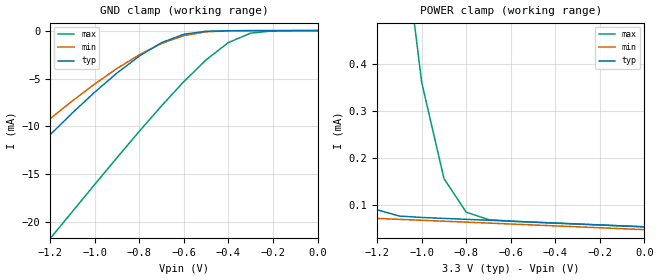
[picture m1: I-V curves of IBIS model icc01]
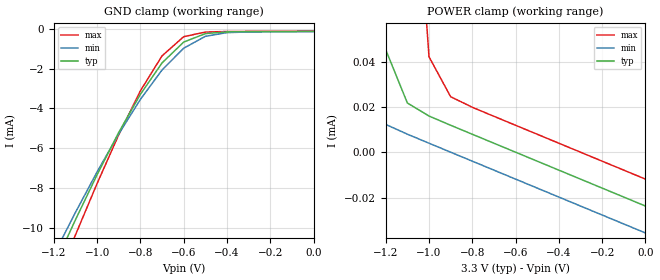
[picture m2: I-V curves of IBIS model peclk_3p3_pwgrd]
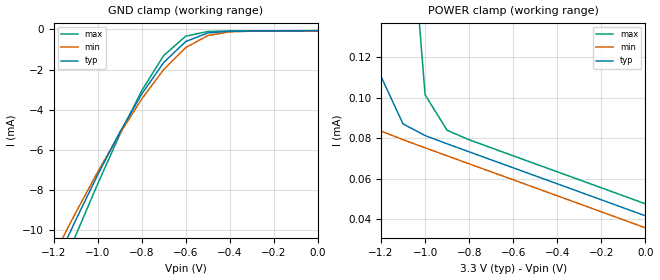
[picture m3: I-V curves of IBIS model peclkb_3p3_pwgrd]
[IBIS ver]   2.1
[File name]   mpc941v2.ibs
[File Rev]   2.2 {April 29, 2002}
[Date]   February 5th, 2002
[Disclaimer]   This information is for modeling purposes only
|   and is not guaranteed.
[Source]   Timing Solutions Operations
[Copyright]   Copyright 2001, Motorola Incorporated,
|   all rights reserved.
[Component]   MPC9413p3
[Manufacturer]   Motorola
[Package]
|   typ   min   max
R_pkg   0.048   .038   0.053
L_pkg   6.045nH   5.084nH   7.950nH
C_pkg   0.813pF   0.560pF   1.157pF
[Pin]   signal_name model_name R_pin L_pin   C_pin
2   OEB   icc01   0.04   0.35nH   0.053pF
3   LVCMOS_CLK   icc01   0.04   0.35nH   0.053pF
4   LVCMOS_CLKSEL   icc01   0.04   0.35nH   0.053pF
6   PCLK   peclk_3p3_pwgrd   0.04   0.35nH   0.053pF
7   PCLK_BAR   peclkb_3p3_pwgrd  0.04   0.35nH   0.053pF
9   Q26   occ01   0.04   0.35nH   0.053pF
10  Q25   occ01   0.04   0.35nH   0.053pF
11  Q24   occ01   0.04   0.35nH   0.053pF
14  Q23   occ01   0.04   0.35nH   0.053pF
15  Q22   occ01   0.04   0.35nH   0.053pF
16  Q21   occ01   0.04   0.35nH   0.053pF
18  Q20   occ01   0.04   0.35nH   0.053pF
19  Q19   occ01   0.04   0.35nH   0.053pF
21  Q18   occ01   0.04   0.35nH   0.053pF
22  Q17   occ01   0.04   0.35nH   0.053pF
23  Q16   occ01   0.04   0.35nH   0.053pF
26  Q15   occ01   0.04   0.35nH   0.053pF
27  Q14   occ01   0.04   0.35nH   0.053pF
28  Q13   occ01   0.04   0.35nH   0.053pF
30  Q12   occ01   0.04   0.35nH   0.053pF
31  Q11   occ01   0.04   0.35nH   0.053pF
33  Q10   occ01   0.04   0.35nH   0.053pF
34  Q09   occ01   0.04   0.35nH   0.053pF
35  Q08   occ01   0.04   0.35nH   0.053pF
38  Q07   occ01   0.04   0.35nH   0.053pF
39  Q06   occ01   0.04   0.35nH   0.053pF
40  Q05   occ01   0.04   0.35nH   0.053pF
42  Q04   occ01   0.04   0.35nH   0.053pF
43  Q03   occ01   0.04   0.35nH   0.053pF
45  Q02   occ01   0.04   0.35nH   0.053pF
46  Q01   occ01   0.04   0.35nH   0.053pF
47  Q00   occ01   0.04   0.35nH   0.053pF
|This section is the 2.5V model data
[Component]   MPC9412p5
[Manufacturer]   Motorola
[Package]
|   typ   min   max
R_pkg   0.048   .038   0.053
L_pkg   6.045nH   5.084nH   7.950nH
C_pkg   0.813pF   0.560pF   1.157pF
[Pin]   signal_name   model_name   R_pin   L_pin   C_pin
2   OEB   icc012p5   0.04   0.35nH   0.053pF
3   LVCMOS_CLK   icc012p5   0.04   0.35nH   0.053pF
4   LVCMOS_CLKSEL   icc012p5   0.04   0.35nH   0.053pF
6   PCLK   peclk_2p5_pwgrd   0.04   0.35nH   0.053pF
7   PCLK_BAR   peclkb_2p5_pwgrd   0.04   0.35nH   0.053pF
9   Q26   occ012p5   0.04   0.35nH   0.053pF
10  Q25   occ012p5   0.04   0.35nH   0.053pF
11  Q24   occ012p5   0.04   0.35nH   0.053pF
14  Q23   occ012p5   0.04   0.35nH   0.053pF
15  Q22   occ012p5   0.04   0.35nH   0.053pF
16  Q21   occ012p5   0.04   0.35nH   0.053pF
18  Q20   occ012p5   0.04   0.35nH   0.053pF
19  Q19   occ012p5   0.04   0.35nH   0.053pF
21  Q18   occ012p5   0.04   0.35nH   0.053pF
22  Q17   occ012p5   0.04   0.35nH   0.053pF
23  Q16   occ012p5   0.04   0.35nH   0.053pF
26  Q15   occ012p5   0.04   0.35nH   0.053pF
27  Q14   occ012p5   0.04   0.35nH   0.053pF
28  Q13   occ012p5   0.04   0.35nH   0.053pF
30  Q12   occ012p5   0.04   0.35nH   0.053pF
31  Q11   occ012p5   0.04   0.35nH   0.053pF
33  Q10   occ012p5   0.04   0.35nH   0.053pF
34  Q09   occ012p5   0.04   0.35nH   0.053pF
35  Q08   occ012p5   0.04   0.35nH   0.053pF
38  Q07   occ012p5   0.04   0.35nH   0.053pF
39  Q06   occ012p5   0.04   0.35nH   0.053pF
40  Q05   occ012p5   0.04   0.35nH   0.053pF
42  Q04   occ012p5   0.04   0.35nH   0.053pF
43  Q03   occ012p5   0.04   0.35nH   0.053pF
45  Q02   occ012p5   0.04   0.35nH   0.053pF
46  Q01   occ012p5   0.04   0.35nH   0.053pF
47  Q00   occ012p5   0.04   0.35nH   0.053pF
| Models and submodels in the file (8): icc01 (Input), peclk_3p3_pwgrd (Input), peclkb_3p3_pwgrd (Input), occ01 (Output), icc012p5 (Input), peclk_2p5_pwgrd (Input), peclkb_2p5_pwgrd (Input), occ012p5 (Output)
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|This is a Model of an CMOS Input with a 50,000 ohm Pull_up at 3.3V
[Model]   icc01
Model_type   Input
Polarity   Non-Inverting
Vmeas=1.5
Vinl=.8
Vinh=2.0
| Variable   typ   min   max
C_comp   5p   5p   5p
[Temperature Range]   27.00   100.00   -45.00
[Power Clamp Reference]   3.30V   3.0V   3.6V
[Gnd Clamp Reference]   0.000V   0.000V   0.000V
[Voltage Range]   3.30V   3.0V   3.6V
[Pulldown Reference]   0.000V   0.000V   0.000V
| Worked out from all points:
|   GND clamp passes 1 mA (typ) near -0.67 V on its own axis
|   POWER clamp passes 1 mA (typ) near -1.50 V on its own axis
[GND_clamp]
|   voltage   I(typ)   I(mim)   I(max)
-3.3V     -64.02mA   -56.37mA   -80.44mA
-1.8V     -25.56mA   -21.69mA   -38.72mA
-1.7V     -23.03mA   -19.5mA    -35.89mA
-1.6V     -20.51mA   -17.33mA   -33.05mA
-1.2V     -10.84mA   -9.179mA   -21.67mA
-1.1V     -8.57mA    -7.315mA   -18.85mA
-900mV    -4.418mA   -3.945mA   -13.24mA
-700mV    -1.251mA   -1.342mA   -7.834mA
-600mV    -381.4uA   -529.5uA   -5.315mA
-400mV    -13.34uA   -24.07uA   -1.246mA
-300mV    -6.264uA   -7.567uA   -268.1uA
1.97fV    -11.82pA   -304.9pA   -5.993uA
[POWER_clamp]
|voltage   I(typ)   I(min)   I(max)
-3.3V     24.4mA     18.52mA    23.82mA
-2.1V     7.098mA    708uA      9.272mA
-2V       5.867mA    235uA      8.195mA
-1.9V     4.703mA    99.99uA    7.152mA
-1.4V     474.5uA    75.62uA    2.627mA
-1.3V     176.1uA    73.63uA    1.907mA
-1.2V     89.81uA    71.64uA    1.272mA
-1.1V     76.66uA    69.65uA    744.2uA
-1V       73.7uA     67.66uA    360.8uA
-900mV    71.64uA    65.67uA    156.3uA
-800mV    69.65uA    63.68uA    84.81uA
1.97fV    53.73uA    47.76uA    53.73uA
|This model is for a Pecl Input at 3.3V
[Model]   peclk_3p3_pwgrd
Model_type   Input
Vmeas=1.5
Vinl=0.8
Vinh=2.0
| Variable   typ   min   max
C_comp   5p   5p   5p
[Temperature Range]   27.00   100.00   -45.00
[Power Clamp Reference]   3.30V   3.00V   3.60V
[Gnd Clamp Reference]   0.000V   0.000V   0.000V
[Voltage Range]   3.30V   3.00V   3.60V
[Pulldown Reference]   0.000V   0.000V   0.000V
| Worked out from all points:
|   GND clamp passes 1 mA (typ) near -0.63 V on its own axis
|   POWER clamp passes 1 mA (typ) near -1.46 V on its own axis
[GND_clamp]
| voltage   I(typ)   I(min)   I(max)
-3.3V     -65.58mA   -61.83mA   -70.36mA
-1.2V     -11.96mA   -11.35mA   -13.02mA
-1.1V     -9.594mA   -9.224mA   -10.36mA
-1V       -7.329mA   -7.188mA   -7.771mA
-900mV    -5.205mA   -5.279mA   -5.323mA
-800mV    -3.291mA   -3.546mA   -3.115mA
-700mV    -1.714mA   -2.069mA   -1.359mA
-600mV    -666.8uA   -975.9uA   -396.7uA
-500mV    -241.6uA   -377.6uA   -163.2uA
-400mV    -155.7uA   -192.2uA   -135.8uA
1.97fV    -130.7uA   -142.6uA   -118.8uA
[POWER_clamp]
| voltage   I(typ)  I(min)  I(max)
-3.3V     27.08mA    21.42mA    33.95mA
-1.5V     1.27mA     194.8uA    3.742mA
-1.4V     587.9uA    51.94uA    2.515mA
-1.3V     181.2uA    19.57uA    1.462mA
-1.2V     45.26uA    12.26uA    649.8uA
-1.1V     21.73uA    7.958uA    178.7uA
-1V       15.97uA    3.969uA    42.13uA
-900mV    11.89uA    5.703nA    24.5uA
-800mV    7.921uA    -3.955uA   19.82uA
1.97fV    -23.76uA   -35.64uA   -11.88uA
|This is a Model of a PECL_BAR Input with a 25,000 ohm Pull_Up at 3.3V
[Model]   peclkb_3p3_pwgrd
Model_type   Input
Vmeas=1.5
Vinl=.8
Vinh=2.0
| Variable   typ   min   max
C_comp   5p   5p   5p
[Temperature Range]   27.00   100.00   -45.00
[Power Clamp Reference]   3.30V   3.00V   3.60V
[Gnd Clamp Reference]   0.000V   0.000V   0.000V
[Voltage Range]   3.30V   3.00V   3.60V
[Pulldown Reference]   0.000V   0.000V   0.000V
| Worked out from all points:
|   GND clamp passes 1 mA (typ) near -0.64 V on its own axis
|   POWER clamp passes 1 mA (typ) near -1.45 V on its own axis
[GND_clamp]
| voltage   I(typ)   I(min)   I(max)
-3.3V     -65.51mA   -61.76mA   -70.3mA
-1.2V     -11.89mA   -11.28mA   -12.96mA
-1.1V     -9.53mA    -9.154mA   -10.3mA
-1V       -7.265mA   -7.118mA   -7.713mA
-900mV    -5.141mA   -5.209mA   -5.265mA
-800mV    -3.227mA   -3.475mA   -3.057mA
-700mV    -1.649mA   -1.999mA   -1.301mA
-600mV    -601.9uA   -905.3uA   -337.6uA
-500mV    -176.4uA   -306.5uA   -103.9uA
-400mV    -90.4uA    -121uA     -76.41uA
1.97fV    -65.34uA   -71.29uA   -59.4uA
[POWER_clamp]
| voltage   I(typ)  I(min)  I(max)
-3.3V     27.15mA    21.49mA    34.01mA
-1.5V     1.335mA    265.9uA    3.8mA
-1.4V     652.9uA    123.2uA    2.573mA
-1.3V     246.4uA    90.85uA    1.52mA
-1.2V     110.6uA    83.55uA    708.8uA
-1.1V     87.07uA    79.24uA    237.9uA
-1V       81.31uA    75.25uA    101.5uA
-900mV    77.23uA    71.29uA    83.9uA
-800mV    73.26uA    67.33uA    79.23uA
1.97fV    41.58uA    35.65uA    47.52uA
